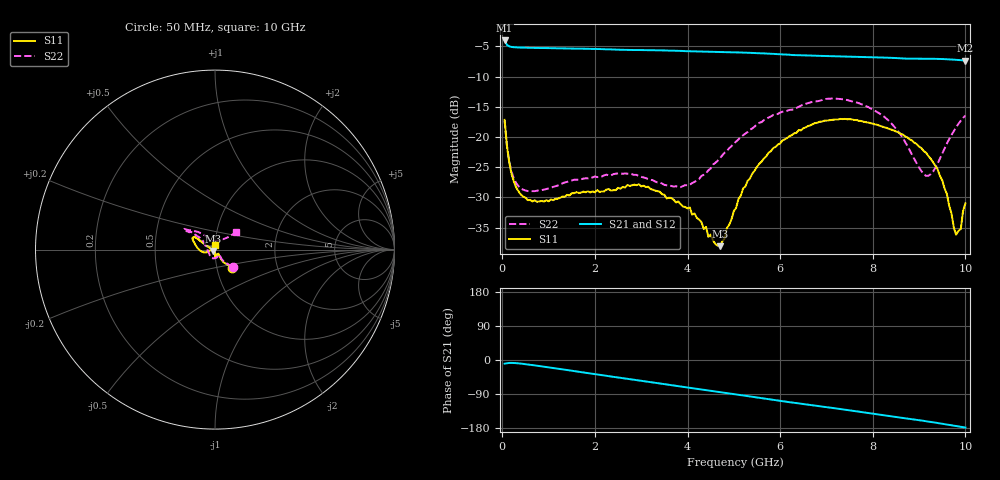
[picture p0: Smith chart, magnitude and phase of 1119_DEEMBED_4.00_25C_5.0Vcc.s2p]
!Hittite Microwave Corp.
!Digital Attenuator/PhaseShifter Rev 1.4.0
!Filename: C:\DATA\DATA\1119_DEEMBED_4.00_25C_5.0Vcc.s2p
!VNA ID: Agilent Technologies,N5224A,MY51441122,A.10.45.03
!Device type:
!2 Port Calibration.
!Temp(C): 25
!Lot Number:
!Serial Number:
!Operator:
!Misc:
!Attenuator:  4.000
# GHZ S DB R 50.0
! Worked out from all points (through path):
!   200 points, 50 MHz to 10 GHz, reference 50 ohm
!   highest |S21| = -4.01 dB at 50 MHz (marker M1); lowest = -7.3 dB at 10 GHz (marker M2)
!   group delay of S21, straight-line fit = 48.3 ps
!   lowest |S11| = -38.1 dB at 4.7 GHz (marker M3), VSWR 1.03, Z = 49 - j0.694 ohm
!   |S11| at or under -10 dB: start of sweep to end of sweep
!   |S22| runs from -29.0 to -13.6 dB; largest |S21 - S12| = 0.0018
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0.05  -17.16 -46.1  -4.01 -9.6  -4.01 -9.6  -17.27 -44.4
0.1  -21.47 -56.5  -4.74 -8.5  -4.74 -8.5  -21.43 -53.8
0.2  -26.13 -57.0  -5.08 -7.6  -5.08 -7.7  -25.77 -53.5
0.4  -29.53 -52.0  -5.19 -9.5  -5.19 -9.6  -28.51 -48.4
0.9  -30.69 -57.4  -5.27 -17.7  -5.27 -17.7  -28.71 -56.6
1.75  -29.04 -80.4  -5.38 -32.8  -5.38 -32.8  -26.88 -79.8
2.75  -28.11 -83.4  -5.58 -50.4  -5.59 -50.5  -26.05 -111.5
3.4  -29.06 -86.6  -5.65 -61.9  -5.65 -61.9  -27.56 -136.6
4.05  -31.67 -85.2  -5.79 -73.4  -5.79 -73.5  -27.90 -173.4
4.45  -36.52 -104.0  -5.89 -80.5  -5.91 -80.5  -25.50 161.2
4.7  -38.07 -145.5  -5.93 -84.8  -5.95 -84.8  -23.50 149.8
5.05  -31.70 166.9  -5.99 -90.9  -6.00 -91.0  -20.75 142.6
5.3  -27.22 157.0  -6.04 -95.4  -6.06 -95.5  -19.15 142.4
5.75  -22.62 151.6  -6.20 -103.5  -6.21 -103.5  -16.77 143.1
6.7  -17.89 148.3  -6.51 -119.3  -6.52 -119.3  -14.17 146.8
7.45  -17.06 153.2  -6.68 -132.0  -6.69 -132.0  -13.88 145.5
8.35  -18.64 163.8  -6.88 -147.8  -6.88 -147.8  -17.33 133.7
9.2  -23.15 -169.2  -7.04 -162.5  -7.05 -162.5  -26.42 90.4
9.5  -27.15 -163.5  -7.08 -168.3  -7.10 -168.3  -22.72 52.3
9.799999  -36.18 156.1  -7.22 -174.3  -7.23 -174.3  -18.38 41.3
9.9  -35.25 111.0  -7.27 -176.3  -7.28 -176.3  -17.30 40.5
10  -30.99 91.1  -7.33 -178.3  -7.34 -178.3  -16.44 40.1
